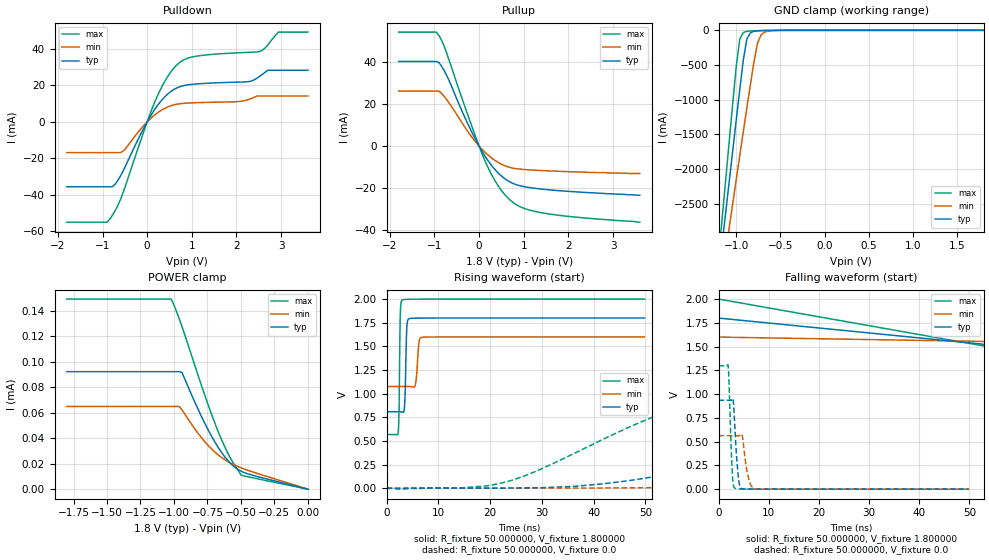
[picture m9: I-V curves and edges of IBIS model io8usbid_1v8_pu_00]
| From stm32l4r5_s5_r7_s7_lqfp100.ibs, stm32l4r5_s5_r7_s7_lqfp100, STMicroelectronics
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|   Model io8usbid_1v8_pu_00
[Model]  io8usbid_1v8_pu_00
Model_type I/O
Polarity   Non-Inverting
Enable   Active-Low
Vinl =   0.540000V
Vinh =   1.260000V
Vmeas =  0.900000V
Cref =   100.000000nF
Rref =   1.000000k
Vref =   1.800000V
C_comp   2.022300pF   2.021100pF   2.049600pF
[Temperature Range]   25.000000   0.125000k   -40.000000
[Pullup Reference]   1.800000V   1.600000V   2.000000V
[Pulldown Reference]   0.0V   0.0V   0.0V
[POWER Clamp Reference]   1.800000V   1.600000V   2.000000V
[GND Clamp Reference]   0.0V   0.0V   0.0V
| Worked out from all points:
|   slope of the pulldown table from 0 to 0.27 V, typ, clamps not added: 26.4 ohm
|   slope of the pullup table from 0 to 0.27 V, typ, clamps not added: 30.1 ohm
|   GND clamp passes 1 mA (typ) near -0.60 V on its own axis
|   rising waveform, R_fixture 50.000000, V_fixture 1.800000: 20-80 % time 251ps typ, 397ps min, 180ps max; typ from 0.81 V to 1.8 V
|   rising waveform, R_fixture 50.000000, V_fixture 0.0: 20-80 % time 65.2ns typ, 114ns min, 35.5ns max; typ from 0.001 V to 0.935 V
|   falling waveform, R_fixture 50.000000, V_fixture 1.800000: 20-80 % time 119ns typ, 161ns min, 92ns max; typ from 1.8 V to 0.81 V
|   falling waveform, R_fixture 50.000000, V_fixture 0.0: 20-80 % time 678ps typ, 984ps min, 517ps max; typ from 0.935 V to 0.001 V
[Pulldown]
|Voltage   I(typ)   I(min)   I(max)
-1.8V     -35.64mA   -16.93mA   -55.1mA
-840mV    -35.64mA   -16.93mA   -53.52mA
-720mV    -34.31mA   -16.93mA   -48.86mA
-540mV    -27.04mA   -16.13mA   -38.89mA
240mV     9.303mA    5.14mA     14.78mA
480mV     15.67mA    8.374mA    25.64mA
720mV     19.18mA    9.883mA    32.46mA
1.14V     20.87mA    10.54mA    36.19mA
2.28V     22.08mA    12.36mA    38.18mA
2.52V     24.96mA    14.18mA    38.63mA
2.94V     28.3mA     14.18mA    49.27mA
3.6V      28.3mA     14.18mA    49.27mA
[Pullup]
|Voltage   I(typ)   I(min)   I(max)
-1.8V     40.48mA    26.32mA    54.53mA
-960mV    40.48mA    26.32mA    54.53mA
-900mV    39.98mA    26.32mA    52.91mA
-780mV    36mA       23.73mA    47.67mA
-240mV    10.08mA    6.588mA    14.1mA
120mV     -4.38mA    -2.702mA   -6.45mA
240mV     -8.143mA   -5.004mA   -12mA
420mV     -12.68mA   -7.723mA   -18.77mA
720mV     -17.48mA   -10.36mA   -26.28mA
1.02V     -19.45mA   -11.2mA    -29.88mA
1.5V      -20.78mA   -11.79mA   -32.25mA
3.6V      -23.5mA    -13.1mA    -36.4mA
[GND_clamp]
|Voltage   I(typ)   I(min)   I(max)
-1.8V     -9.895A    -9.296A    -9.457A
-1.2V     -3.533A    -3.902A    -3.274A
-1.16V    -3.082A    -3.55A     -2.716A
-1.12V    -2.631A    -3.198A    -2.159A
-1.08V    -2.182A    -2.848A    -1.604A
-1V       -1.289A    -2.15A     -512mA
-960mV    -849.4mA   -1.803A    -123.8mA
-920mV    -422.4mA   -1.459A    -30.79mA
-880mV    -123.7mA   -1.118A    -13.63mA
-760mV    -6.32mA    -185mA     -5.692mA
-680mV    -2.569mA   -25.43mA   -2.907mA
1.8V      0A         0A         0A
[POWER_clamp]
|Voltage   I(typ)   I(min)   I(max)
-1.8V     92.32uA    64.98uA    149.4uA
-1.02V    92.32uA    64.98uA    149.4uA
-960mV    92.32uA    64.98uA    133.7uA
-940mV    91.68uA    62.28uA    127.8uA
-800mV    58.29uA    41.17uA    83.14uA
-700mV    38.06uA    29.69uA    53.4uA
-640mV    28.2uA     24.57uA    37.82uA
-600mV    22.83uA    21.83uA    28.76uA
-560mV    18.54uA    19.56uA    21uA
-500mV    14.23uA    16.82uA    11.13uA
-400mV    10.56uA    13.15uA    8.664uA
0V        0A         0A         0A
[Ramp]
| variable   typ   min   max
dV/dt_r  0.56071/65.15866n   0.33710/0.11418u   0.77863/35.46512n
dV/dt_f  0.59414/66.69548n   0.31416/0.11610u   0.85869/35.03815n
R_load = 50.000000
[Rising Waveform]
R_fixture= 50.000000
V_fixture= 1.800000
V_fixture_min= 1.600000
V_fixture_max= 2.000000
|time   V(typ)   V(min)   V(max)
0s        809.8mV    1.076V     568.8mV
2.202ns   809.8mV    1.076V     579.4mV
2.402ns   809.8mV    1.076V     855.9mV
2.603ns   809.7mV    1.076V     1.798V
3.003ns   806mV      1.076V     1.99V
3.504ns   911mV      1.077V     1.996V
3.904ns   1.719V     1.077V     1.997V
4.304ns   1.792V     1.076V     1.998V
6.807ns   1.799V     1.595V     1.999V
49.85ns   1.8V       1.6V       2V
[Rising Waveform]
R_fixture= 50.000000
V_fixture= 0.0
V_fixture_min= 0.0
V_fixture_max= 0.0
|time   V(typ)   V(min)   V(max)
0s        726.2uV    1.152mV    482.7uV
22.82ns   3.295mV    2.596mV    64.72mV
42.04ns   49.46mV    4.288mV    523.9mV
63.66ns   246.9mV    17.07mV    982.9mV
79.28ns   415.6mV    41.15mV    1.158V
98.5ns    593.6mV    95.26mV    1.243V
121.3ns   739.6mV    176.4mV    1.278V
159.8ns   867.5mV    308.8mV    1.294V
251.1ns   929.6mV    494.8mV    1.298V
598.2ns   935.3mV    563.1mV    1.298V
[Falling Waveform]
R_fixture= 50.000000
V_fixture= 1.800000
V_fixture_min= 1.600000
V_fixture_max= 2.000000
|time   V(typ)   V(min)   V(max)
0s        1.8V       1.6V       2V
150.2ns   1.017V     1.47V      598.5mV
300.3ns   823.1mV    1.139V     569.6mV
450.5ns   811mV      1.089V     568.9mV
750.8ns   809.7mV    1.077V     568.8mV
14.86us   809.8mV    1.076V     568.8mV
[Falling Waveform]
R_fixture= 50.000000
V_fixture= 0.0
V_fixture_min= 0.0
V_fixture_max= 0.0
|time   V(typ)   V(min)   V(max)
0s        935.3mV    563.1mV    1.298V
1.902ns   935.3mV    563.1mV    1.304V
2.703ns   946.8mV    563.1mV    193.1mV
2.903ns   943.6mV    563.1mV    54.99mV
3.303ns   586.7mV    563mV      8.665mV
4.004ns   99.27mV    562.8mV    2.544mV
4.705ns   5.495mV    566.4mV    1.762mV
5.806ns   1.186mV    152.1mV    1.574mV
7.107ns   794.5uV    4.738mV    1.508mV
49.85ns   726.2uV    1.152mV    482.7uV
